(* Logix 5000 AddOnInstructionDefinition export ACS_INCREMENTAL_MOVE; software revision 20.01 *)

ADD_ON_INSTRUCTION ACS_INCREMENTAL_MOVE   (* revision 2.0, vendor Tolomatic, Inc *)
// Move to a position relative to current position
VAR_INPUT
   Distance : REAL; {required}   // Distance to Travel (Positive or Negative)
   Acceleration : REAL; {required}   // Trajectory Acceleration
   Deceleration : REAL; {required}   // Trajectory Deceleration
   Velocity : REAL; {required}   // Trajectory Constance Velocity
   Force : REAL; {required}   // Force Limit (Percent)
END_VAR
VAR_IN_OUT
   DriveMoveSelect : SINT; {required}   // ACS.O.MOVESELECT
   DriveTargetAcc : REAL; {required}   // ACS.O.TARGET_0_ACC
   DriveTargetDec : REAL; {required}   // ACS.O.TARGET_0_DEC
   DriveTargetForce : REAL; {required}   // ACS.O.TARGET_0_FORCE
   DriveTargetMotionType : DINT; {required}   // ACS.O.TARGET_0_MOTION_TYPE
   DriveTargetPos : REAL; {required}   // ACS.O.TARGET_0_POS
   DriveTargetVel : REAL; {required}   // ACS.O.TARGET_0_VEL
END_VAR
VAR
   AbsDistance : REAL; {access None}   // Absolute Value of Distance Input
END_VAR

ROUTINE Logic   (* ladder *)
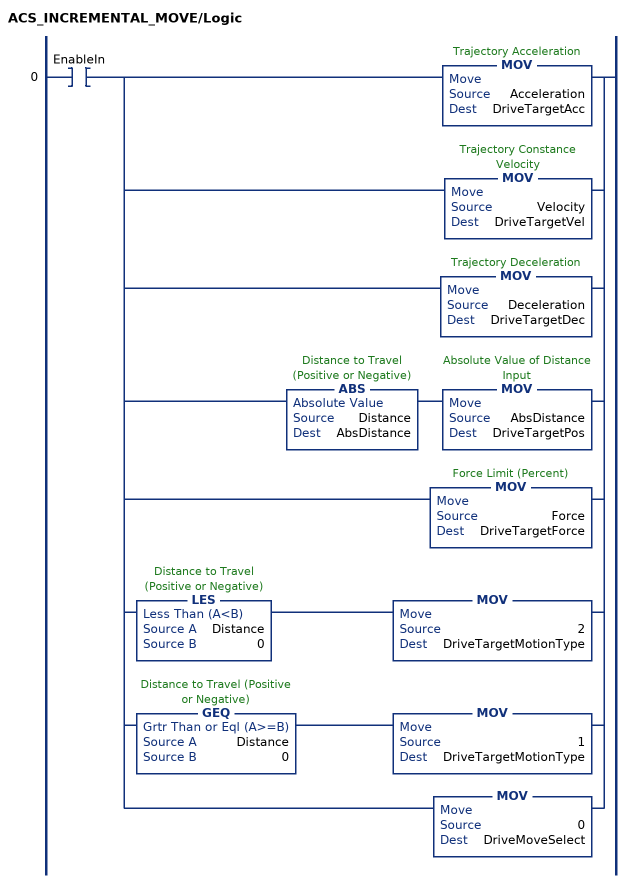
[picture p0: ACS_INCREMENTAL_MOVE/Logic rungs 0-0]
   0: XIC(EnableIn)[MOV(Acceleration,DriveTargetAcc) ,MOV(Velocity,DriveTargetVel) ,MOV(Deceleration,DriveTargetDec) ,ABS(Distance,AbsDistance) MOV(AbsDistance,DriveTargetPos) ,MOV(Force,DriveTargetForce) ,LES(Distance,0) MOV(2,DriveTargetMotionType) ,GEQ(Distance,0) MOV(1,DriveTargetMotionType) ,MOV(0,DriveMoveSelect) ];
END_ROUTINE
END_ADD_ON_INSTRUCTION
